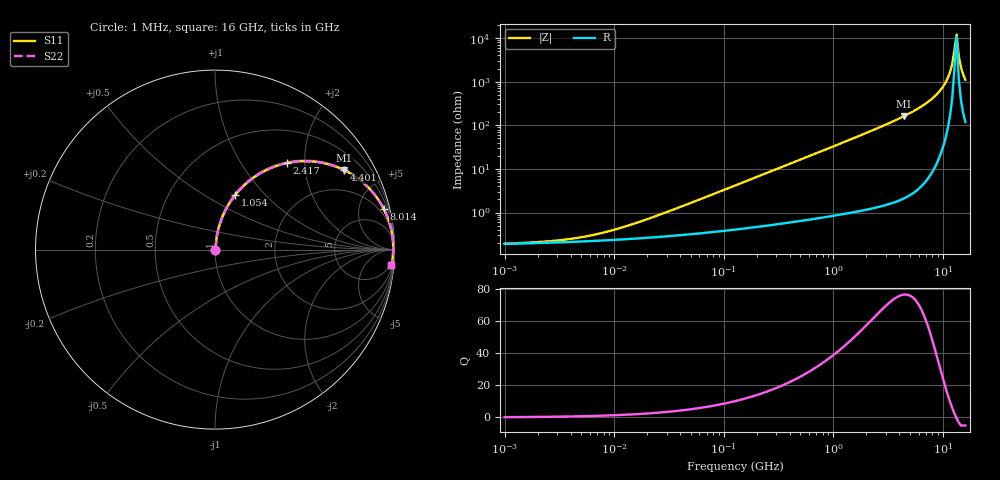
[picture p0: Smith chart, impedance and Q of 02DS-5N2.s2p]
# MHz S MA R 50
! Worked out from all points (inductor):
!   211 points, 1 MHz to 16 GHz, reference 50 ohm
!   read as one part in series: L = 5.2 nH near 26.39 MHz
!   highest Q = 76.6 at 4.401 GHz (marker M1), where L = 5.85 nH
!   self-resonance near 12.71 GHz
!   S11 on the Smith chart (normalised r, x): 1 MHz: 1.00, +0.00; 1.054 GHz: 1.02, +0.69; 2.417 GHz: 1.03, +1.63; 4.401 GHz: 1.04, +3.24; 8.014 GHz: 1.17, +8.30; 16 GHz: 3, -22
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1  0.001934 9.7  0.9981 -0.0  0.9981 -0.0  0.001934 9.7
2.63276  0.00221 22.8  0.998 -0.0  0.998 -0.0  0.00221 22.8
5.25662  0.00277 38.1  0.9978 -0.1  0.9978 -0.1  0.00277 38.1
10.9906  0.004307 56.1  0.9976 -0.2  0.9976 -0.2  0.004307 56.1
26.3872  0.009033 71.6  0.9972 -0.5  0.9972 -0.5  0.009033 71.6
132.458  0.04326 82.1  0.995 -2.5  0.995 -2.5  0.04326 82.1
318.018  0.103 81.1  0.9893 -5.9  0.9893 -5.9  0.103 81.1
664.915  0.2115 75.9  0.9705 -12.2  0.9705 -12.2  0.2115 75.9
1054.3  0.3252 69.6  0.9376 -19.0  0.9376 -19.0  0.3252 69.6
1596.39  0.4642 61.2  0.8767 -27.7  0.8767 -27.7  0.4642 61.2
2417.22  0.628 50.2  0.7684 -38.9  0.7684 -38.9  0.628 50.2
3187.38  0.7367 41.8  0.666 -47.4  0.666 -47.4  0.7367 41.8
4401.2  0.8458 31.5  0.5227 -57.7  0.5227 -57.7  0.8458 31.5
6077.26  0.925 21.5  0.367 -67.7  0.367 -67.7  0.925 21.5
8013.56  0.9676 13.5  0.2332 -75.3  0.2332 -75.3  0.9676 13.5
10090.8  0.9869 7.1  0.1243 -80.4  0.1243 -80.4  0.9869 7.1
11587.3  0.9921 3.4  0.06021 -80.7  0.06021 -80.7  0.9921 3.4
12134  0.9928 2.2  0.03913 -78.3  0.03913 -78.3  0.9928 2.2
13305.8  0.9927 -0.2  0.008228 28.0  0.008228 28.0  0.9927 -0.2
13933.5  0.9919 -1.4  0.02626 71.4  0.02626 71.4  0.9919 -1.4
14590.9  0.9906 -2.7  0.04703 77.2  0.04703 77.2  0.9906 -2.7
16000  0.9865 -5.1  0.08923 78.8  0.08923 78.8  0.9865 -5.1
